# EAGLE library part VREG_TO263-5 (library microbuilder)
TO263-5 Linear Voltage Regulators LD29300xx - 3A LDO (Vf: 0.4V@3A, 0.2V@1A) - Digikey: 3.3V - 497-3475-1-ND LD29300P2MTR - 3A LDO Adjustable - Digikey: 497-7780-1-ND, Mouser: 511-LD29300P2MTR
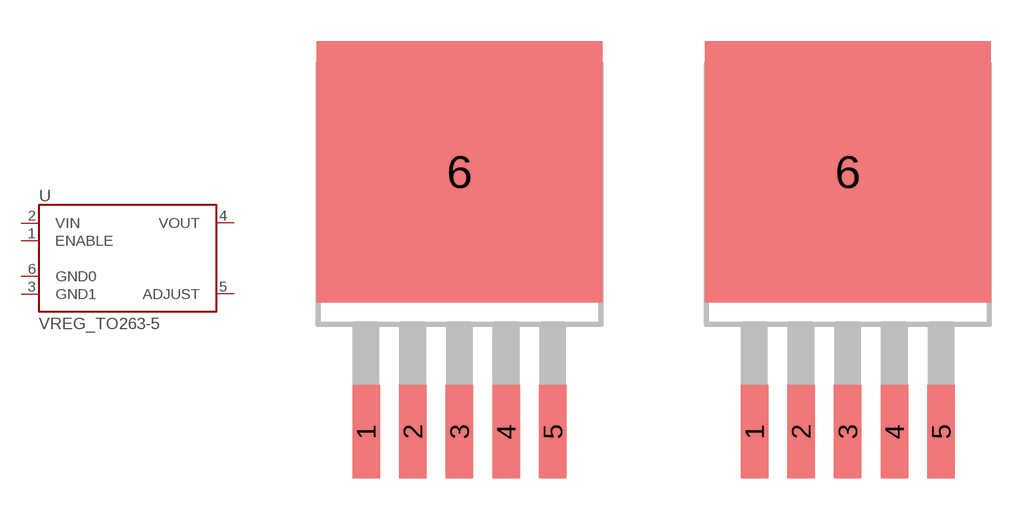
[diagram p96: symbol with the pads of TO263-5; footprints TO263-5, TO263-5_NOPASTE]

Designator prefix U

## VREG_TO263-5  [TO263-5]
1  ENABLE
2  VIN
3  GND1
4  VOUT
5  ADJUST
6  GND0

## VREG_TO263-5NOPASTE  [TO263-5_NOPASTE]
Pads as for TO263-5

## Footprint TO263-5 (pad centres in mm)
Warning: Part outline is approximative
smd 1 x 3.4: 1 -3.4,-7.875; 2 -1.7,-7.875; 3 0,-7.875; 4 1.7,-7.875; 5 3.4,-7.875
smd 10.414 x 9.525: 6 0,1.595

## Footprint TO263-5_NOPASTE (pad centres in mm)
smd 1 x 3.4: 1 -3.4,-9.145; 2 -1.7,-9.145; 3 0,-9.145; 4 1.7,-9.145; 5 3.4,-9.145
smd 10.414 x 9.525: 6 0,0.325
